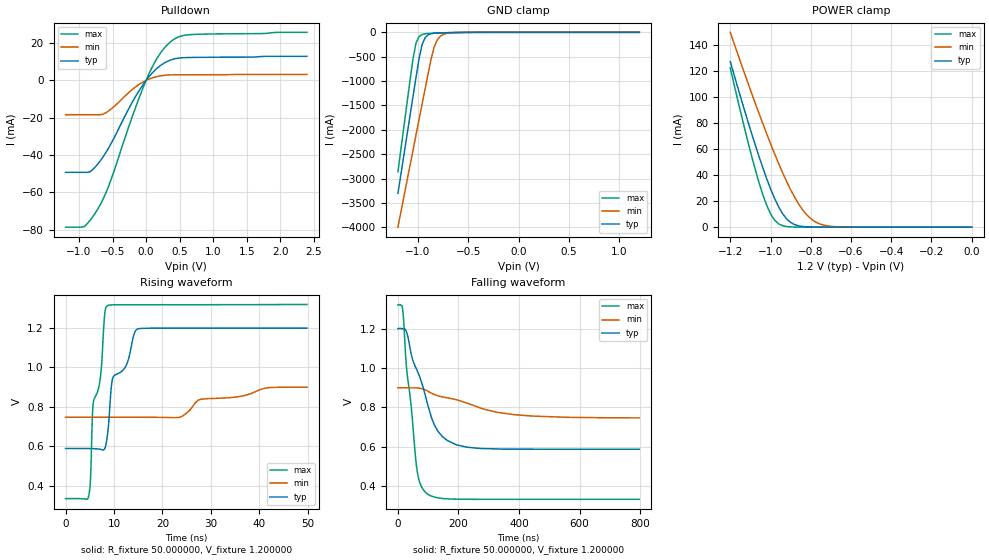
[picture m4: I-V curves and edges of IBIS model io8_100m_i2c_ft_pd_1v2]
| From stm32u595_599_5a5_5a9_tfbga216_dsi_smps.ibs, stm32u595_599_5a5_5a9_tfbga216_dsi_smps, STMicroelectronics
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|   Model io8_100m_i2c_ft_pd_1v2
[Model]  io8_100m_i2c_ft_pd_1v2
Model_type I/O_open_drain
Polarity   Non-Inverting
Enable   Active-Low
Vinl =   0.360000V
Vinh =   0.840000V
Vmeas =  0.500000V
Cref =   50.000000pF
Rref =   100.000000
Vref =   0.600000V
C_comp   2.954600pF   2.884400pF   3.002700pF
[Temperature Range]   25.000000   0.140000k   -40.000000
[Pullup Reference]   1.200000V   0.900000V   1.320000V
[Pulldown Reference]   0.0V   0.0V   0.0V
[POWER Clamp Reference]   1.200000V   0.900000V   1.320000V
[GND Clamp Reference]   0.0V   0.0V   0.0V
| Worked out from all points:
|   slope of the pulldown table from 0 to 0.18 V, typ, clamps not added: 25.7 ohm
|   GND clamp passes 1 mA (typ) near -0.51 V on its own axis
|   POWER clamp passes 1 mA (typ) near -0.86 V on its own axis
|   rising waveform, R_fixture 50.000000, V_fixture 1.200000: 20-80 % time 4.46ns typ, 13ns min, 2.41ns max; typ from 0.588 V to 1.2 V
|   falling waveform, R_fixture 50.000000, V_fixture 1.200000: 20-80 % time 78.1ns typ, 207ns min, 36ns max; typ from 1.2 V to 0.588 V
[Pulldown]
|Voltage   I(typ)   I(min)   I(max)
-1.2V     -49.24mA   -18.34mA   -78.58mA
-920mV    -49.24mA   -18.34mA   -78.22mA
-840mV    -48.98mA   -18.34mA   -75.14mA
-720mV    -44.76mA   -18.34mA   -68.87mA
-560mV    -36.26mA   -16.38mA   -56.73mA
-200mV    -11.29mA   -4.684mA   -18.8mA
0V        0A         0A         -10fA
160mV     6.399mA    2.052mA    11.64mA
360mV     10.87mA    2.957mA    20.57mA
480mV     11.93mA    3.021mA    23.25mA
640mV     12.29mA    3.041mA    24.48mA
2.4V      12.92mA    3.23mA     25.77mA
[GND_clamp]
|Voltage   I(typ)   I(min)   I(max)
-1.2V     -3.305A    -3.998A    -2.862A
-1.05V    -1.316A    -2.418A    -539.3mA
-1.02V    -921mA     -2.103A    -218.8mA
-990mV    -539.5mA   -1.788A    -87.45mA
-960mV    -252.2mA   -1.474A    -44.37mA
-930mV    -110.5mA   -1.16A     -30.33mA
-870mV    -28.04mA   -549.1mA   -21.1mA
-840mV    -18.44mA   -305.6mA   -18.29mA
-810mV    -13.92mA   -159.7mA   -15.75mA
-780mV    -11.24mA   -82.36mA   -13.39mA
-600mV    -2.986mA   -4.279mA   -3.072mA
1.2V      30.28uA    18.17uA    37.27uA
[POWER_clamp]
|Voltage   I(typ)   I(min)   I(max)
-1.2V     127mA      149.4mA    122.2mA
-1.12V    84.97mA    114mA      70.27mA
-1.06V    55.51mA    88.42mA    35.67mA
-1.02V    37.63mA    72.04mA    17.17mA
-1V       29.51mA    64.13mA    10.3mA
-960mV    15.69mA    48.99mA    2.571mA
-900mV    3.624mA    28.77mA    182.8uA
-840mV    490.7uA    13.24mA    11.35uA
-800mV    116.8uA    6.532mA    1.77uA
-740mV    13.2uA     1.723mA    109.1nA
-620mV    167.3nA    79.35uA    0A
0V        0A         17.84nA    0A
[Ramp]
| variable   typ   min   max
dV/dt_r  0.36632/4.44892n   91.26600m/13.03294n 0.59111/2.40596n
dV/dt_f  0.36698/77.99434n   91.41000m/0.20683u  0.59153/35.97865n
R_load = 50.000000
[Rising Waveform]
R_fixture= 50.000000
V_fixture= 1.200000
V_fixture_min= 0.900000
V_fixture_max= 1.320000
|time   V(typ)   V(min)   V(max)
0s        587.8mV    746.8mV    333.5mV
4.805ns   587.7mV    746.8mV    350.5mV
5.105ns   587.5mV    746.8mV    414.9mV
5.706ns   586.9mV    746.8mV    819mV
7.107ns   584.2mV    746.8mV    934.3mV
8.008ns   584.2mV    746.8mV    1.253V
8.509ns   632.4mV    746.8mV    1.311V
9.71ns    943.4mV    746.8mV    1.318V
14.81ns   1.195V     746.7mV    1.318V
49.85ns   1.199V     899.4mV    1.319V
[Falling Waveform]
R_fixture= 50.000000
V_fixture= 1.200000
V_fixture_min= 0.900000
V_fixture_max= 1.320000
|time   V(typ)   V(min)   V(max)
0s        1.199V     899.4mV    1.319V
16.02ns   1.199V     899.7mV    1.293V
28.83ns   1.181V     899.3mV    994.3mV
43.24ns   1.075V     899.1mV    812.9mV
64.06ns   984.9mV    898.5mV    472.3mV
94.49ns   837.2mV    885.3mV    364.5mV
137.7ns   668.2mV    856.6mV    339.6mV
222.6ns   599.7mV    824.9mV    333.8mV
382.8ns   587.9mV    763.3mV    333.5mV
797.6ns   587.8mV    746.8mV    333.5mV
